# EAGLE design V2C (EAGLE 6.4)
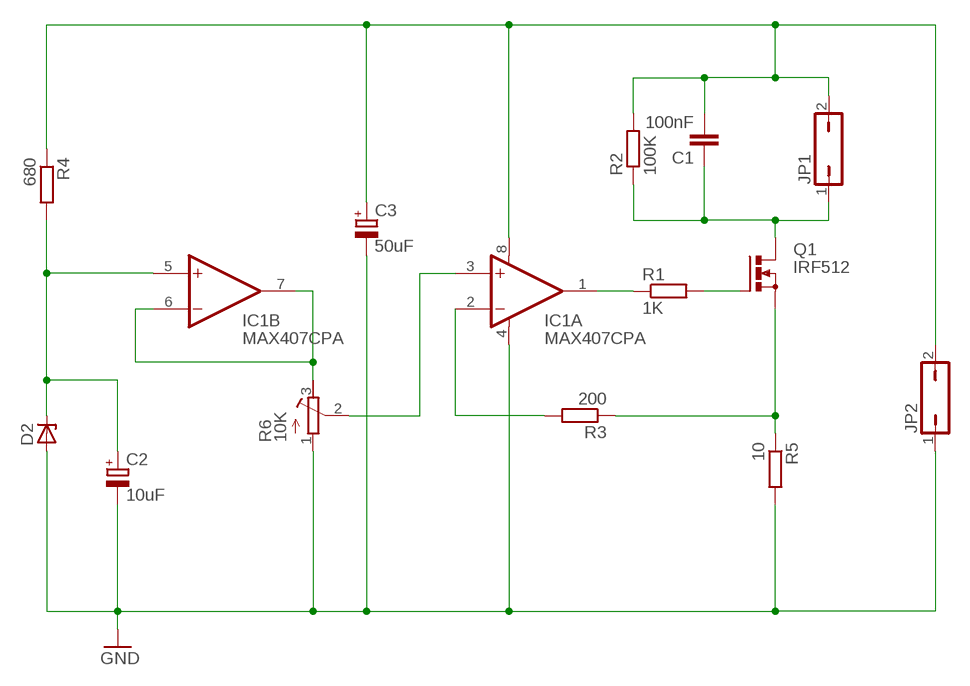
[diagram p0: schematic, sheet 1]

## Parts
C1  100nF  C-EU050-030X075  [C050-030X075]
C2  10uF  CPOL-EUE2.5-6  [E2,5-6]
C3  50uF  CPOL-EUE2.5-6  [E2,5-6]
D2  ZENER-DIODEDO35Z10  [DO35Z10]
IC1  MAX407CPA  [DIL08]
JP1  JP1Q  [JP1]
JP2  JP1Q  [JP1]
Q1  IRF512  [TO220BV]
R1  1K  R-EU_0204/7  [0204/7]
R2  100K  R-EU_0204/7  [0204/7]
R3  200  R-EU_0204/7  [0204/7]
R4  680  R-EU_0204/7  [0204/7]
R5  10  R-EU_0207/12  [0207/12]
R6  10K  R-TRIMM64W  [RTRIM64W]

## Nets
GND: C2.- C3.- D2.A IC1.4(A:V-) JP2.1 R5.2 R6.1(A)
N$2: C2.+ D2.C IC1.5(B:+IN) R4.2
N$3: C1.2 C3.+ IC1.8(A:V+) JP1.2 JP2.2 R2.2 R4.1
N$6: IC1.6(B:-IN) IC1.7(B:OUT) R6.3(E)
N$7: IC1.3(A:+IN) R6.2(S)
N$8: IC1.1(A:OUT) R1.1
N$9: Q1.G R1.2
N$10: Q1.S R3.1 R5.1
N$11: IC1.2(A:-IN) R3.2
N$12: C1.1 JP1.1 Q1.D R2.1

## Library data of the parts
C1 = rcl:C-EU: CAPACITOR, European symbol
C2 C3 = rcl:CPOL-EU: POLARIZED CAPACITOR, European symbol
D2 = diode:ZENER-DIODE: Z-Diode
IC1 = maxim:MAX407CPA: OP AMP; MPN: MAX407CPA+; OC_FARNELL: unknown; OC_NEWARK: 03M8833
JP1 JP2 = jumper:JP1Q: JUMPER
Q1 = transistor-power:IRF512: N-CHANNEL MOS FET
R1-R5 = rcl:R-EU_: RESISTOR, European symbol
R6 = rcl:R-TRIMM: Trimm resistor

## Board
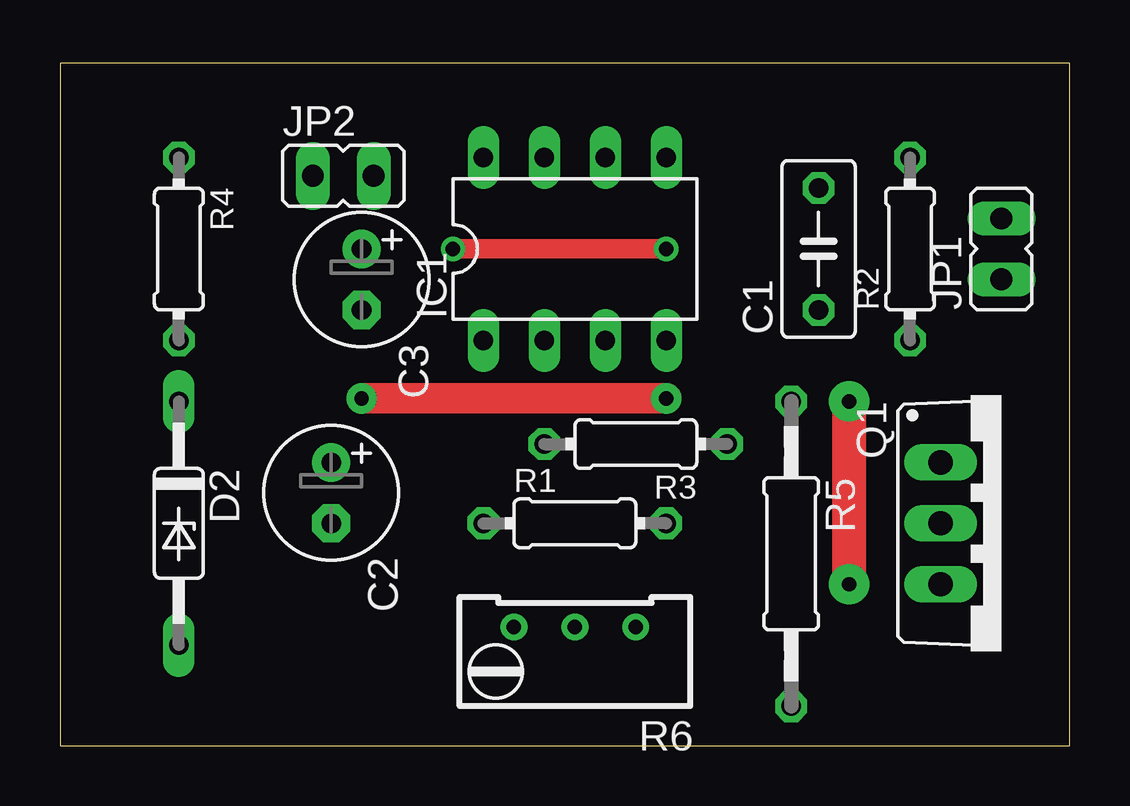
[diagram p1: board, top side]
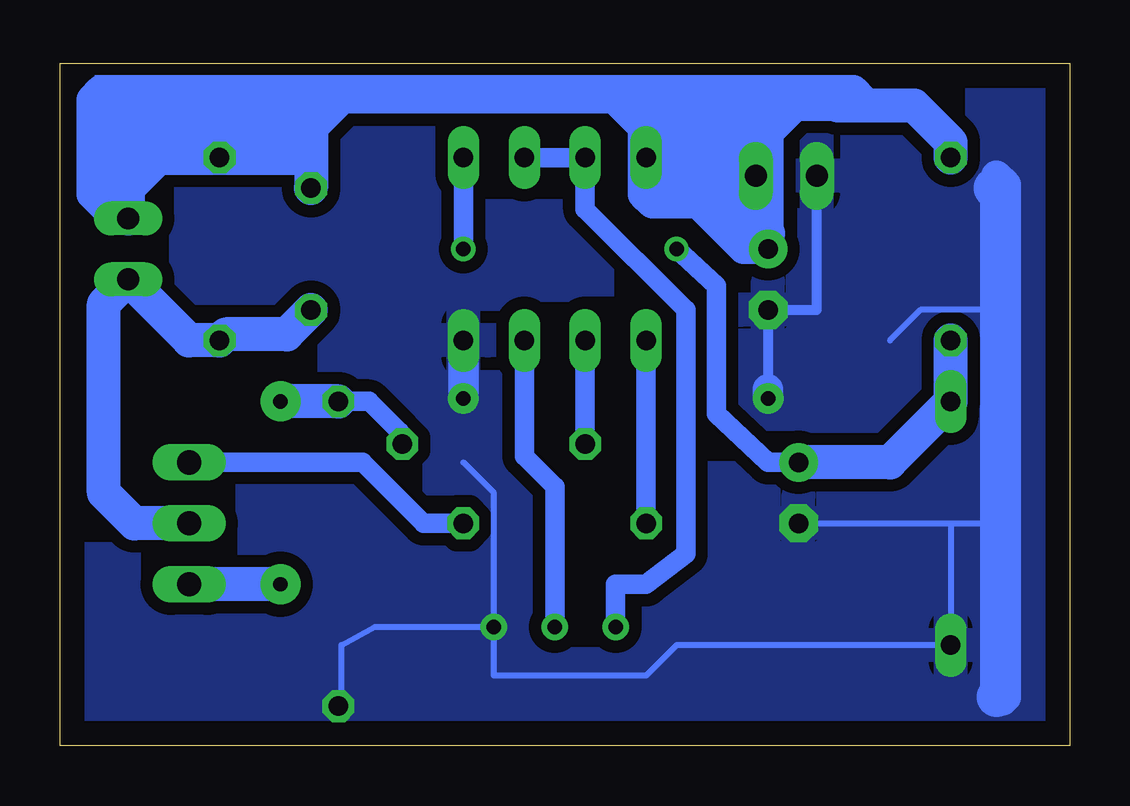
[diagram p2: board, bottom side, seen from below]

Size 42.09 x 28.44 mm. Coordinates in mm from the lower left corner, seen from the top.
Outline: 0,0 42.09,0 42.09,28.44 0,28.44 0,0
Copper layers (1*16): Top 0.035mm / dielectric 1.5mm / Bottom 0.035mm
Design rules "default *": minimum track width 10mil, minimum drill 24mil, track to track 20mil, track to pad 20mil, pad to pad 20mil, via to via 20mil, smd to smd 20mil, copper to edge 40mil, drill to drill 8mil, minimum pad ring 10mil, minimum via ring 8mil, stop-mask expansion 4mil, vias tented up to drill 0mil, thermal gap 10mil

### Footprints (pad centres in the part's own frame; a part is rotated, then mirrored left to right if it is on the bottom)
C050-030X075 = drill 0.813 octagon: 1 -2.54,0; 2 2.54,0
E2,5-6 = drill 0.813 pad 1.6: + -1.27,0 | drill 0.813 pad 1.6 octagon: - 1.27,0
DO35Z10 = drill 0.813 long: A 5.08,0; C -5.08,0
DIL08 = drill 0.813 long: 1 -3.81,-3.81; 2 -1.27,-3.81; 3 1.27,-3.81; 4 3.81,-3.81; 5 3.81,3.81; 6 1.27,3.81; 7 -1.27,3.81; 8 -3.81,3.81
JP1 = drill 0.914 long: 1 0,-1.27; 2 0,1.27
TO220BV = drill 1.016 long: D 0,-2.54; G -2.54,-2.54; S 2.54,-2.54
0204/7 = drill 0.813 octagon: 1 -3.81,0; 2 3.81,0
0207/12 = drill 0.813 octagon: 1 -6.35,0; 2 6.35,0
RTRIM64W = drill 0.61: 1 1.27,-2.54; 2 1.27,0; 3 1.27,2.54

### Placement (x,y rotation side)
C1  31.62,20.7 90 top
C2  11.3,10.54 270 top
C3  12.57,19.43 270 top
D2  4.95,9.27 270 top
IC1  21.46,20.7 0 top
JP1  39.24,20.7 0 top
JP2  11.81,23.75 270 top
Q1  39.24,9.27 270 top
R1  21.46,9.27 0 top
R2  35.43,20.7 90 top
R3  24,12.57 180 top
R4  4.95,20.7 270 top
R5  30.48,8 270 top
R6  21.46,3.68 90 top

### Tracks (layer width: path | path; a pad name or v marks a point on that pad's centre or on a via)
GND  (via drill 0.6 pad 1.27)
  Top 1.27: v12.57,14.48 v25.27,14.48
  Bottom 0.254: R6.1 28.96,4.95 30.35,4.19 30.35,1.65 R5.2 | 25.27,11.81 24,10.54 R6.1 | 4.95,9.27 D2.A 16.38,4.19 17.65,2.92 24,2.92 R6.1 | C2.- 4.95,9.27 | 7.49,16.89 6.22,18.16 3.68,18.16 2.41,16.89 2.41,9.27 4.95,9.27
  Bottom 0.406: JP2.1 10.54,18.16 C3.- 12.57,14.86
  Bottom 1.27: 3.05,23.75 2.67,23.37 2.67,2.03 2.79,1.91 | 12.57,14.86 v12.57,14.48 | v25.27,14.48 IC1.4
  Bottom 1.676: 3.17,23.24 2.92,22.99 2.92,2.16 3.05,2.03
  pour Bottom: -1.14,29.34 43.31,29.21 43.31,0 -1.14,0.13
N$1
  Bottom 1.27: 8.64,26.92 9.02,27.3 16.76,27.3
N$2  (via drill 0.6)
  Top 0.813: v16.38,20.7 v25.27,20.7
  Bottom 0.813: C2.+ 12.57,11.81 14.73,13.84 14.73,19.18 v16.38,20.7 | v25.27,20.7 IC1.5
  Bottom 1.422: R4.2 D2.C 7.49,11.81 C2.+
N$3
  Bottom 0.254: 15.11,27.05 16.38,27.05
  Bottom 1.27: 17.65,25.4 17.65,25.65 19.05,27.05 | C3.+ 13.59,20.7 15.49,22.61 17.4,22.61 17.78,22.99
  Bottom 1.422: 12.83,27.05 10.03,27.05 9.65,26.67 6.48,26.67 4.95,25.15 R4.1 | 12.83,27.05 16.38,27.05 | 16.38,27.05 17.65,25.78 17.65,25.4 IC1.8 | 16.38,27.05 19.05,27.05 30.35,27.05 31.62,25.78 31.62,24.51 | 31.62,24.51 C1.2 | JP1.2 39.24,23.24 37.97,24.51 R2.2 31.62,24.51 | 12.83,27.05 13.08,26.8 JP2.2 12.83,23.5 12.83,21.59 12.57,21.34 C3.+
N$4
  Bottom 1.27: 12.83,24.89 12.83,25.27 11.43,26.67
N$5
  Bottom 1.27: 12.7,21.59 12.95,21.59 14.35,22.99 17.53,22.99 17.65,23.11
N$6
  Bottom 0.813: IC1.6 IC1.7 20.19,22.35 16,18.16 16,8 17.65,6.73 18.92,6.73 R6.3
N$7
  Bottom 0.813: R6.2 21.46,10.79 22.73,12.06 IC1.3
N$8
  Bottom 0.813: IC1.1 R1.1
N$9
  Bottom 0.813: R1.2 26.92,9.27 29.46,11.81 Q1.G
N$10  (via drill 0.6 pad 1.68)
  Top 1.422: v32.89,14.35 v32.89,6.73
  Bottom 0.813: R3.1 27.94,13.08 29.21,14.35 R5.1
  Bottom 1.422: R5.1 v32.89,14.35 | v32.89,6.73 Q1.S
N$11
  Bottom 0.813: IC1.2 R3.2
N$12
  Bottom 1.422: C1.1 32.64,17.14 35.18,17.14 R2.1 36.7,16.89 JP1.1 40.26,18.41 40.26,10.54 38.99,9.27 Q1.D
N$13
  Bottom 1.27: 39.75,27.3 40.39,27.3 40.77,26.92 40.77,22.99 40.01,22.23 40.01,26.8
(copper drawn outside any net)
  shapes: Bottom area x5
